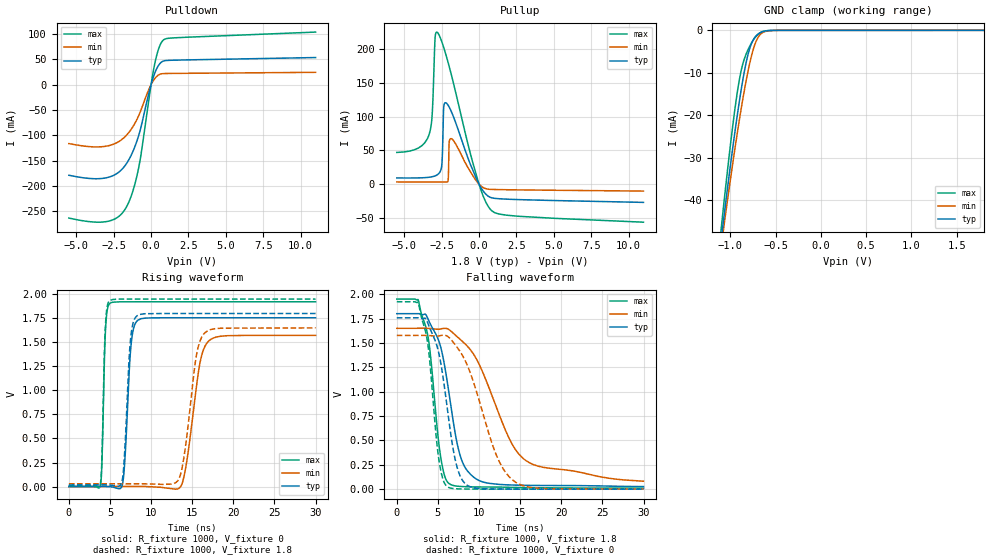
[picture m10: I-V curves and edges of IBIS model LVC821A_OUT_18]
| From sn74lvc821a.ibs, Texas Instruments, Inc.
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[Model]   LVC821A_OUT_18
Model_type  3-state
Enable   Active-Low
Vref =   0
Rref =   1000
Cref =   30p
Vmeas =   0.9
| variable   typ   min   max
C_comp   6.95pF   6.31pF   7.90pF
| C_pullup   8.57pF   7.75pF   9.35pF
| C_pulldown   11.76pF   7.71pF   18.48pF
| C_tri-state   6.95pF   6.31pF   7.90pF
[Temperature Range]   40   100   -40
| Ambient temperature   25   85   -40
[Voltage range]   1.8   1.65   1.95
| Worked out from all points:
|   slope of the pulldown table from 0 to 0.27 V, typ, clamps not added: 11.1 ohm
|   slope of the pullup table from 0 to 0.27 V, typ, clamps not added: 27.1 ohm
|   GND clamp passes 1 mA (typ) near -0.70 V on its own axis
|   rising waveform, R_fixture 1000, V_fixture 0: 20-80 % time 629ps typ, 1.45ns min, 338ps max; typ from 0 V to 1.76 V
|   falling waveform, R_fixture 1000, V_fixture 1.8: 20-80 % time 2.21ns typ, 4.85ns min, 1.42ns max; typ from 1.8 V to 0.026 V
|   rising waveform, R_fixture 1000, V_fixture 1.8: 20-80 % time 615ps typ, 1.36ns min, 335ps max; typ from 0.017 V to 1.8 V
|   falling waveform, R_fixture 1000, V_fixture 0: 20-80 % time 1.9ns typ, 3.65ns min, 1.31ns max; typ from 1.76 V to 0.001 V
[GND Clamp]
| LVC821A_OUT_18
|   Voltage   I(typ)   I(min)   I(max)
-5.5V     -1.089A    -967.7mA   -1.248A
-1.11V    -50.55mA   -52.05mA   -48.2mA
-1.08V    -45.27mA   -47.3mA    -42.15mA
-1.065V   -42.66mA   -44.96mA   -39.18mA
-975mV    -27.71mA   -31.36mA   -22.53mA
-890mV    -15.13mA   -19.57mA   -10.34mA
-855mV    -10.68mA   -15.16mA   -7.294mA
-795mV    -4.82mA    -8.521mA   -4.08mA
-745mV    -2.127mA   -4.295mA   -2.202mA
-695mV    -897.7uA   -1.679mA   -937.2uA
-535mV    -23.89uA   -40.3uA    -11.5uA
1.8V      40.7pA     294.2pA    39.61pA
[Pulldown]
| LVC821A_OUT_18
|   Voltage   I(typ)   I(min)   I(max)
-5.5V     -178.8mA   -116.4mA   -263.3mA
-2.905V   -183.2mA   -121mA     -269.7mA
-2.16V    -172.7mA   -112.5mA   -260mA
-1.625V   -154.8mA   -99.18mA   -240mA
-1.195V   -130.5mA   -81.96mA   -207.7mA
-815mV    -98.94mA   -60.37mA   -161.6mA
-630mV    -78.26mA   -46.61mA   -129.3mA
30mV      3.177mA    1.703mA    5.775mA
280mV     25.08mA    13.03mA    45.92mA
555mV     40.14mA    19.8mA     74.55mA
840mV     46.53mA    21.61mA    88.21mA
11V       53.22mA    24.07mA    103.4mA
[Pullup]
| LVC821A_OUT_18
|   Voltage   I(typ)   I(min)   I(max)
-5.5V     9.186mA    3.268mA    46.91mA
-3.34V    10.21mA    3.178mA    73.37mA
-3.145V   10.92mA    3.169mA    98.96mA
-2.945V   12.17mA    3.16mA     213.7mA
-2.82V    13.46mA    3.154mA    225mA
-2.495V   27.06mA    3.137mA    211.1mA
-2.365V   112.5mA    3.129mA    202.5mA
-2.22V    120.4mA    3.123mA    191.9mA
-2.07V    116.8mA    4.84mA     180.2mA
-1.865V   108mA      67.36mA    163.1mA
845mV     -20.22mA   -7.78mA    -39.27mA
11V       -26.98mA   -10.24mA   -56.27mA
[Ramp]
| LVC821A_OUT_18
| variable   typ   min   max
dV/dt_r   1.07/6.41E-10   0.96/1.48E-09   1.16/3.50E-10
dV/dt_f   1.06/2.21E-09   0.94/4.84E-09   1.16/1.42E-09
R_load = 1000
[Rising Waveform]
| LVC821A_OUT_18
R_fixture =   1000
C_fixture =   0
L_fixture =   0
V_fixture =   0
V_fixture_min = 0
V_fixture_max = 0
|   Time   V(typ)   V(min)   V(max)
0s        461.3pV    823.2pV    246pV
3.845ns   676.7uV    155.6uV    14.78mV
4.465ns   477.8uV    379uV      1.645V
5.005ns   -1.41mV    459uV      1.907V
6.555ns   39.72mV    487.9uV    1.921V
7.535ns   1.449V     498.8uV    1.922V
8.375ns   1.729V     524uV      1.922V
13.67ns   1.756V     10.07mV    1.922V
17.09ns   1.756V     1.52V      1.922V
29.99ns   1.756V     1.573V     1.922V
[Falling Waveform]
| LVC821A_OUT_18
R_fixture =   1000
C_fixture =   0
L_fixture =   0
V_fixture =   1.8
V_fixture_min = 1.65
V_fixture_max = 1.95
|   Time   V(typ)   V(min)   V(max)
0s        1.8V       1.65V      1.95V
2.645ns   1.8V       1.651V     1.932V
3.89ns    1.728V     1.649V     1.515V
5.06ns    1.532V     1.64V      506mV
6.35ns    983.8mV    1.637V     57.6mV
7.82ns    314.6mV    1.528V     27.68mV
9.96ns    90.29mV    1.29V      22.75mV
13.66ns   43.76mV    521.9mV    19.06mV
15.68ns   39.57mV    294.3mV    16.02mV
29.99ns   26.4mV     81.74mV    10.55mV
[Rising Waveform]
| LVC821A_OUT_18
R_fixture =   1000
C_fixture =   0
L_fixture =   0
V_fixture =   1.8
V_fixture_min = 1.65
V_fixture_max = 1.95
|   Time   V(typ)   V(min)   V(max)
0s        16.7mV     28.54mV    9.957mV
3.83ns    17.24mV    28.72mV    29.6mV
4.43ns    17.02mV    28.89mV    1.648V
4.98ns    15.39mV    28.92mV    1.936V
6.515ns   79.86mV    28.8mV     1.95V
7.465ns   1.5V       28.72mV    1.95V
8.27ns    1.775V     28.66mV    1.95V
13.4ns    1.8V       82.92mV    1.95V
16.6ns    1.8V       1.604V     1.95V
29.99ns   1.8V       1.65V      1.95V
[Falling Waveform]
| LVC821A_OUT_18
R_fixture =   1000
C_fixture =   0
L_fixture =   0
V_fixture =   0
V_fixture_min = 0
V_fixture_max = 0
|   Time   V(typ)   V(min)   V(max)
0s        1.758V     1.577V     1.923V
2.645ns   1.758V     1.577V     1.904V
3.795ns   1.699V     1.576V     1.473V
4.84ns    1.481V     1.571V     496.8mV
6.13ns    836.4mV    1.57V      26.53mV
7.105ns   302.3mV    1.481V     4.74mV
8.135ns   73.66mV    1.349V     1.688mV
12.05ns   1.739mV    360.7mV    428.7uV
14.17ns   825.2uV    88.12mV    622.3uV
29.99ns   596.6uV    1.11mV     106.8uV
